VAR_GLOBAL
	
//datapoints SLAVE -> MASTER (monitoring direction)
	(* Input *)

	(* Output *)
	
	(* Memory *)

	(* Data *)
		(*Single Points*)
			// bSlaveToMaster 
			bSlaveToMaster			: BOOL;		// obj addr: 10 - M_SP_NA_1
			nSIQ_bSlaveToMaster		: BYTE;		// data value and qualifier
			eSPI_bSlaveToMaster		: E_IEC870_5_101SPI; // data value as enum type
			nQDS_bSlaveToMaster		: BYTE; // data qualifier
			
		(*Bitstrings*)
			// nBitstring
			nBitstring 				: DWORD;	// obj addr: 11 - M_BO_NA_1;
			nQDS_nBitstring			: BYTE;		// data qualifier
		
		(*Measurement Value*)
			// nMeasurementValue - scaled value
			nMeasurementValue		: INT;		// obj addr: 12 - M_ME_NB_1
			nQDS_nMeasurementValue 	: BYTE;		// data qualifier
			
			// fMeasurementValue - short floating point value 
			fMeasurementValue 		: REAL;		// obj addr: 13 - M_ME_NC_1
			nQDS_fMeasurementValue	: BYTE;		// data qualifier
			
		
//datapoints MASTER -> SLAVE (control direction)
	(* Input *)

	(* Output *)
	
	(* Memory *)

	(* Data*)
		(*Single Commands*)
			// bMasterToSlave 
			bMasterToSlave			: BOOL;		// obj addr: 101 - C_SC_NA_1
			nSCO_bMasterToSlave		: BYTE;		// command value and qualifier
			eSCS_bMasterToSlave		: E_IEC870_5_101SCS; // data value as enum type
			eQU_bMasterToSlave		: E_IEC870_5_101QU; // command qualifier
			

//other variables

END_VAR
